VAR_GLOBAL
   nSetBaudrate               : UINT := 10417; // Für Rx-Delay-Berechnung
   (* I/O variables for EL6001 terminal acting as Master*)
   COMin_EL6001_MASTER AT %I* : EL6inData22B;(* linked to the EL6001 in the TwinCAT System Manager *)
   COMout_EL6001_MASTER AT %Q*: EL6outData22B;(* linked to the EL6001 in the TwinCAT System Manager *)
   RxBuffer_MASTER            : ComBuffer;(* Receive data buffer; used with all receive function blocks *)
   TxBuffer_MASTER            : ComBuffer;(* Transmit data buffer; used with all receive function blocks *)
END_VAR
